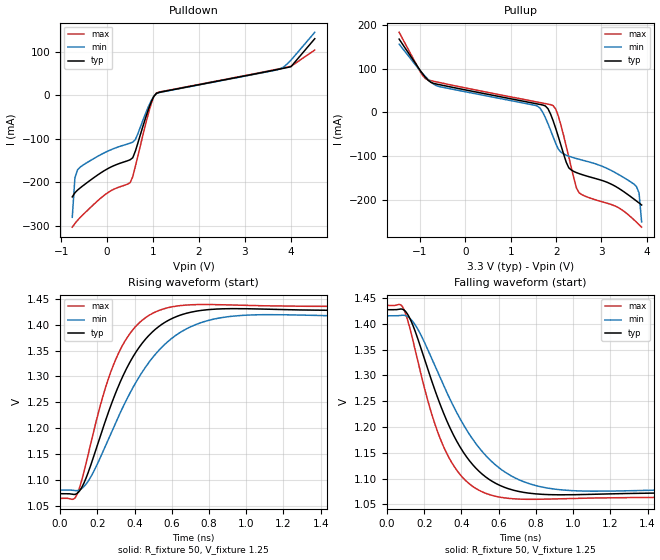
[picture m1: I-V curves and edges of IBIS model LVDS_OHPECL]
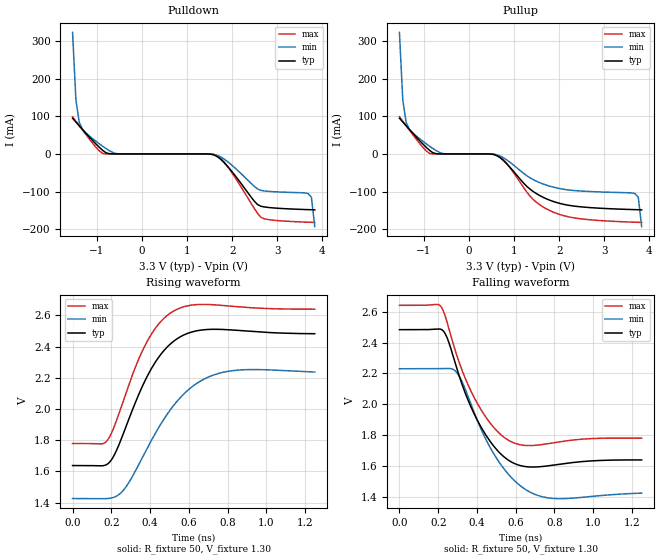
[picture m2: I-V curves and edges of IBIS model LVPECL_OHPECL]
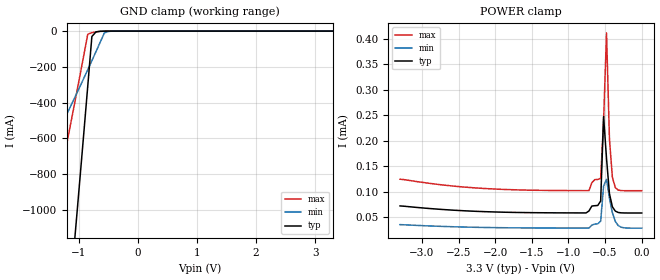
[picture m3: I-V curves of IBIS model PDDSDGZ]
|   This file is an IBIS representation of the   |
|   Integrated Device Technology Inc   |
|   IDT82P33714A   |
|   Synchronous Equipment Timing   |
|   Source for Synchronous Ethernet   |
[IBIS Ver]   4.1
[File name]   82p33714a.ibs
[File Rev]   0.5
|Rev 0.5
|08 Dec 2014
|Allegro Model Editor parse results, File passed: 0 errors, 33 warnings
|Rev 0.4
|06 Dec 2014
|pin 56 model name and pin name is NC because the pad is not bonded out
|Rev 0.3
|05 Dec 2014
|Added pin 73 as GND (ePad connection)
|Rev 0.2
|04 Dec 2014
|Updated pins 45 and 46
|Rev 0.1
|03 Dec 2014
|Original Model
[Date]   03 DEC 2014
[Source]   Originated at Integrated Device Technology, Inc.
[Notes]
No notes
[Disclaimer]
IDT hereby grants the user of this IBIS model a non-exclusive,
non-transferable license to use this IBIS model under the following terms.
Before using this IBIS model, the user should read this license.
If the user does not accept these terms,  the IBIS model should be
returned to IDT within 30 days.
   The user is granted this license only to use the IBIS model and
is not granted rights to sell, load, rent, lease or license the IBIS
model in whole or in part, or in modified form to anyone other than
user. User may modify the IBIS model to suit its specific
applications but rights to derivative works and such modifications
shall belong to IDT.
   This IBIS model is provided on an "AS IS" basis and IDT makes
absolutely no warranty with respect to the information contained
herein. IDT DISCLAIMS AND CUSTOMER WAIVES ALL WARRANTIES, EXPRESS
OR IMPLIED, INCLUDING WARRANTIES OF MERCHANTABILITY OR FITNESS FOR
A PARTICULAR PURPOSE. The entire risk as to quality and performance
is with the Customer. ACCORDINGLY, IN NO EVENT SHALL THE COMPANY BE
LIABLE FOR ANY DAMAGES, WHETHER IN CONTRACT OR TORT,INCLUDING ANY
LOST PROFITS OR OTHER INCIDENTAL, CONSEQUENTIAL, EXEMPLARY, OR
PUNITIVE DAMAGES ARISING OUT OF THE USE OR APPLICATION OF THE IBIS
model provided in this package. Further, IDT reserves the right to
make changes without notice to any product herein to improve
reliability, function, or design. IDT does not convey any license
under patent rights or any other intellectual property rights,
including those of third parties.
   IDT is not obligated to provide maintenance or support
for the licensed IBIS model.
[Copyright] Copyright 2014 by Integrated Device Technology, Inc.
[Component]   IDT82P33714A
[Manufacturer] Integrated Device Technology, Inc.
[Package]
|NLG 72
|   typ   min   max
R_pkg   0.14662   0.14662   0.14662
L_pkg   2.064e-9   2.064e-9   2.064e-9
C_pkg   3.399e-12   3.399e-12   3.399e-12
[Pin]   signal_name   model_name   R_pin   L_pin   C_pin
1   VC2   NC   159.1129532e-3  2.330616742e-9  290.6011e-15
2   VDDA   POWER   80.55656693e-3  1.627074523e-9  368.4314e-15
3   VDDA   POWER   82.37314399e-3  1.61436763e-9   359.8344e-15
4   VDDA   POWER   83.90273432e-3  1.632152529e-9  365.4028e-15
5   VDDA   POWER   88.16928499e-3  1.691978222e-9  379.0725e-15
6   OSCI   PDIDGZ   146.7372238e-3  2.417572968e-9  292.6019e-15
7   XO_FREQ0/LOS0   PDDSDGZ   133.245742e-3   2.24699185e-9   280.7049e-15
8   XO_FREQ1/LOS1   PDDSDGZ   124.3227716e-3  2.089820262e-9  264.6841e-15
9   XO_FREQ2/LOS2   PDDSDGZ   119.3648461e-3  1.952561307e-9  249.2576e-15
10   VDDA   POWER   67.96352653e-3  1.277137683e-9  316.527e-15
11   VDDA   POWER   124.3606471e-3  1.803394983e-9  258.8162e-15
12   VDDA   POWER   45.40697553e-3  1.045816154e-9  381.861e-15
13   VC1   NC   122.5820275e-3  1.79486331e-9   251.4324e-15
14   TMS   PDUSDGZ   117.199996e-3   1.881836464e-9  243.7828e-15
15   TRSTB   PDUSDGZ   117.9505235e-3  1.959346923e-9  249.952e-15
16   TCK   PDDSDGZ   124.0105416e-3  2.055224639e-9  260.0248e-15
17   TDI   PDUSDGZ   132.6063283e-3  2.195081403e-9  275.8995e-15
18   TDO   PDT02DGZ   139.0580983e-3  2.375490982e-9  254.5569e-15
19   VSSAO   GND   81.99029019e-3  1.941331922e-9  317.2106e-15
20   VDDAO   POWER   73.85343737e-3  1.662854677e-9  366.3893e-15
21   OUT4_POS   PECL_LVDS04 121.7311063e-3  1.941431983e-9  266.714e-15
22   OUT4_NEG   PECL_LVDS04 107.5226543e-3  1.73548545e-9   231.1601e-15
23   VSSAO   GND   55.50550232e-3  1.238142672e-9  269.1671e-15
24   VDDAO   POWER   51.03037114e-3  1.120699481e-9  265.15e-15
25   OUT3_POS   PECL_LVDS04 88.13552011e-3  1.429561675e-9  207.5597e-15
26   OUT3_NEG   PECL_LVDS04 84.21161109e-3  1.379390516e-9  197.1123e-15
27   VDDDO   POWER   46.76944028e-3  998.9182167e-9  232.0838e-15
28   OUT2   PDO08CDG   86.16174582e-3  1.377671438e-9  199.8731e-15
29   VDDDO   POWER   47.51781649e-3  996.4207054e-9  245.1067e-15
30   OUT1   PDO08CDG   92.05055036e-3  1.515185344e-9  202.4479e-15
31   IN1_POS   lvdspecl_rx 86.6701243e-3   1.443347965e-9  198.2298e-15
32   IN1_NEG   lvdspecl_rx 93.91076143e-3  1.549324015e-9  215.2678e-15
33   IN2_POS   lvdspecl_rx 104.444426e-3   1.718046615e-9  233.5331e-15
34   IN2_NEG   lvdspecl_rx 116.8021523e-3  1.932360839e-9  258.363e-15
35   IN3_POS   lvdspecl_rx 131.5182922e-3  2.179307422e-9  291.0504e-15
36   IN3_NEG   lvdspecl_rx 141.9756831e-3  2.439789828e-9  273.2442e-15
37   IN5   PDDSDGZ   140.0551623e-3  2.412978327e-9  247.8168e-15
38   IN4_POS   lvdspecl_rx 126.4230008e-3  2.142248554e-9  254.6755e-15
39   IN4_NEG   lvdspecl_rx 119.9314187e-3  2.029050584e-9  247.6935e-15
40   VDDD   POWER   117.0922381e-3  1.990478433e-9  243.7891e-15
41   IN6   PDDSDGZ   61.39234119e-3  1.45567977e-9   290.6114e-15
42   VDDD_1_8   POWER   62.64670293e-3  1.428642413e-9  280.9995e-15
43   FRSYNC_8K_1PPS   PDO04CDG   125.5118157e-3  2.091755546e-9  248.7724e-15
44   MFRSYNC_2K_1PPS   PDO04CDG   118.5182609e-3  2.032772465e-9  241.1773e-15
45   MPU_MODE0/I2CM_SDA   PDU02SDGZ   118.7248552e-3  2.079337927e-9  237.1947e-15
46   MPU_MODE1/I2CM_SCL   PDU02SDGZ   116.1434147e-3  2.040116685e-9  240.7992e-15
47   SDI/I2C_AD2/UART_RX   PDDSDGZ   113.9184373e-3  2.005672797e-9  243.2646e-15
48   CLKE/I2C_AD1   PDDSDGZ   114.7639065e-3  2.023372275e-9  243.911e-15
49   CS/I2C_AD0   PDUSDGZ   119.2670929e-3  2.063087241e-9  249.1366e-15
50   SCLK/I2C_SCL   PDDSDGZ   125.4625035e-3  2.170317538e-9  259.0128e-15
51   SDO/I2C_SDA/UART_TX   PDU02SDGZ   134.5129774e-3  2.297443305e-9  272.3048e-15
52   RSTB   PDUSDGZ   144.9448535e-3  2.469905075e-9  278.2184e-15
53   VDDD_1_8   POWER   73.18502347e-3  1.697897064e-9  321.7456e-15
54   DPLL3_LOCK   PDO02CDG   73.30587215e-3  1.805509644e-9  286.9406e-15
55   DPLL1_LOCK   PDO02CDG   131.2037581e-3  2.269971476e-9  249.9768e-15
56   NC   NC
57   INT_REQ   PDT02DGZ   111.9942974e-3  1.823787365e-9  244.1426e-15
58   MS/SL   PDUSDGZ   54.06374355e-3  1.208304195e-9  279.0375e-15
59   LOS3   PDDSDGZ   91.44979742e-3  1.501013847e-9  210.5244e-15
60   OUT10   PDO08CDG   88.55779602e-3  1.462256672e-9  201.0622e-15
61   OUT9   PDO08CDG   83.69588131e-3  1.389134256e-9  199.3806e-15
62   VDDD   POWER   47.94070401e-3  993.0254377e-9  238.4781e-15
63   OUT8   PDO08CDG   88.97797819e-3  1.387693063e-9  197.6827e-15
64   VDDDO   POWER   50.19081992e-3  1.056276793e-9  240.4795e-15
65   OUT7   PDO08CDG   91.25440696e-3  1.457201564e-9  206.4251e-15
66   VDDDO   POWER   55.34448696e-3  1.15702755e-9   257.2621e-15
67   OUT6_NEG   PECL_LVDS04 100.1273738e-3  1.588127846e-9  221.0412e-15
68   OUT6_POS   PECL_LVDS04 113.6333223e-3  1.762765097e-9  250.6782e-15
69   VDDAO   POWER   70.67244584e-3  1.428806307e-9  324.875e-15
70   OUT5_NEG   PECL_LVDS04 124.2699555e-3  1.951978145e-9  261.0113e-15
71   OUT5_POS   PECL_LVDS04 142.9203716e-3  2.168494279e-9  305.0693e-15
72   VDDAO   POWER   93.00146904e-3  1.898111852e-9  344.1775e-15
73   VSSAO   GND   81.99029019e-3  1.941331922e-9  317.2106e-15
[Diff Pin]   inv_pin   vdiff   tdelay_typ   tdelay_min   tdelay_max
|Inputs
 31   32   100mV   NA   NA   NA
 33   34   100mV   NA   NA   NA
 35   36   100mV   NA   NA   NA
 38   39   100mV   NA   NA   NA
|Outputs
 25   26   NA   0   0   0
 21   22   NA   0   0   0
 71   70   NA   0   0   0
 68   67   NA   0   0   0
[Model Selector] PECL_LVDS04
LVDS_OHPECL   3.3V LVDS Output Driver
LVPECL_OHPECL   3.3V LVPECL Output Driver
| Models and submodels in the file (11): LVDS_OHPECL (Output), LVPECL_OHPECL (Output_ECL), PDDSDGZ (Input), PDO08CDG (Output), PDO04CDG (Output), PDO02CDG (Output), PDUSDGZ (Input), lvdspecl_rx (Input), PDT02DGZ (3-state), PDU02SDGZ (I/O), PDIDGZ (Input)
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[Model]   LVDS_OHPECL
Model_type   Output
Polarity   Non-Inverting
|   typ   min   max
C_comp   2pF   1.5pF   2.5pF
Vmeas = 1.25V
Rref = 50
Cref = 0
Vref = 1.25V
|   typ   min   max
[Voltage range]   3.3V   3.135V   3.465V
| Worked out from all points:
|   slope of the pulldown table from 0 to 0.495 V, typ, clamps not added: 23.6 ohm
|   slope of the pullup table from 0 to 0.495 V, typ, clamps not added: 49.3 ohm
|   rising waveform, R_fixture 50, V_fixture 1.25: 20-80 % time 245ps typ, 304ps min, 193ps max; typ from 1.07 V to 1.43 V
|   falling waveform, R_fixture 50, V_fixture 1.25: 20-80 % time 245ps typ, 304ps min, 193ps max; typ from 1.43 V to 1.07 V
[Pulldown]
|Voltage   I (typ)   I (min)   I (max)
|Note, modeling breaks down at 250mA and above.  This is well beyond the functional   |
|operating range of the device.  Should this scenario occur, catastrophic failure and   |
|possible damage to the device and/or board is of higher concern than the I-V curve   |
|behavior.  The IBIS checker will flag currents in excess of 10A with warnings.  Lines   |
|with currents in excess of 0.35 A have been commented out.  The points still remain|
|available to the user if the user desires to use them.   |
|-2.84000e+00   -5.30688e+01   -4.60169e+01   -6.49561e+01
|-2.38000e+00   -4.07182e+01   -3.57367e+01   -4.91647e+01
|-1.92000e+00   -2.83653e+01   -2.54540e+01   -3.33724e+01
|-1.46000e+00   -1.60091e+01   -1.51695e+01   -1.75745e+01
|-1.00000e+00   -3.65295e+00   -4.88655e+00   -1.77315e+00
|-9.90000e-01   -3.38442e+00   -4.66309e+00   -1.42972e+00
|-9.32644e-01   -1.84442e+00   -3.38153e+00   -4.05588e-01
|-8.75287e-01   -5.22833e-01   -2.10025e+00   -3.26469e-01
|-8.17931e-01   -2.67482e-01   -8.21699e-01   -3.12033e-01
-760.6mV  -233mA     -279.7mA   -302.3mA
-703.2mV  -223.5mA   -189.3mA   -293.9mA
-645.9mV  -217.5mA   -171.1mA   -286.7mA
-14.94mV  -170mA     -129.6mA   -225.5mA
501.3mV   -147.9mA   -109.9mA   -200.6mA
558.6mV   -143.4mA   -107.5mA   -186.7mA
616mV     -128mA     -101.6mA   -163.1mA
960.1mV   -15.71mA   -12.63mA   -19.86mA
1.075V    4.077mA    3.606mA    4.898mA
3.771V    60mA       60.11mA    60.87mA
4.01V     65.35mA    80.22mA    66.12mA
4.528V    129.4mA    144mA      103.5mA
| 5.04600e+00   2.59994e-01   1.76348e+00   2.05360e-01
| 5.56400e+00   3.32161e+00   4.50935e+00   1.54088e+00
| 6.08200e+00   6.62030e+00   7.25691e+00   5.75525e+00
| 6.60000e+00   9.92114e+00   1.00065e+01   9.97217e+00
[Pullup]
|Voltage   I (typ)   I (min)   I (max)
|Note, modeling breaks down at 250mA and above.  This is well beyond the functional   |
|operating range of the device.  Should this scenario occur, catastrophic failure and   |
|possible damage to the device and/or board is of higher concern than the I-V curve   |
|behavior.  The IBIS checker will flag currents in excess of 10A with warnings.  Lines   |
|with currents in excess of 0.35 A have been commented out.  The points still remain|
|available to the user if the user desires to use them.   |
|-2.84000e+00   6.99085e+00   6.68991e+00   7.57174e+00
|-2.38000e+00   4.06132e+00   4.25024e+00   3.82819e+00
|-1.92000e+00   1.13336e+00   1.81188e+00   3.20303e-01
-1.46V    167mA      155.6mA    182.5mA
-875.3mV  79.39mA    80.95mA    76.56mA
-588.5mV  63.59mA    59.29mA    68.52mA
1.591V    19.2mA     14.2mA     23.52mA
1.82V     8.437mA    -25.7mA    18.9mA
1.935V    -19.25mA   -55.77mA   15.52mA
2.05V     -55.57mA   -83.85mA   -8.737mA
2.279V    -126.2mA   -99.7mA    -101.3mA
2.509V    -139.6mA   -106.9mA   -183.4mA
3.771V    -201.8mA   -168.9mA   -250.1mA
3.828V    -206.4mA   -183.2mA   -255.8mA
3.885V    -211.1mA   -249.6mA   -261.5mA
| 3.94264e+00   -2.16138e-01   -6.40744e-01   -2.67350e-01
| 4.00000e+00   -2.22049e-01   -1.86978e+00   -2.73217e-01
| 4.01000e+00   -2.23263e-01   -2.09313e+00   -2.74250e-01
| 4.52800e+00   -9.77564e+00   -1.36708e+01   -3.93552e+00
| 5.04600e+00   -2.36907e+01   -2.52521e+01   -2.17292e+01
| 5.56400e+00   -3.76023e+01   -3.68312e+01   -3.95166e+01
| 6.08200e+00   -5.15104e+01   -4.84070e+01   -5.72987e+01
| 6.60000e+00   -6.54191e+01   -5.99802e+01   -7.50835e+01
[Ramp]
|   typ   min   max
dV/dt_r   0.215/0.251n   0.204/0.312n   0.226/0.197n
dV/dt_f   0.858/0.18n   0.851/0.206n   0.863/0.152n
R_load =   50.0000
[Rising Waveform]
R_fixture = 50
V_fixture = 1.25   |Vcc_typ
V_fixture_min = 1.25 |Vcc_min
V_fixture_max = 1.25 |Vcc_max
C_fixture = 0.0p
| Time   typ   min   max
0s        1.073V     1.08V      1.064V
76.08ps   1.071V     1.079V     1.063V
114.1ps   1.084V     1.082V     1.096V
222.2ps   1.191V     1.148V     1.252V
296.3ps   1.266V     1.209V     1.331V
386.4ps   1.335V     1.275V     1.388V
496.5ps   1.386V     1.336V     1.422V
666.7ps   1.421V     1.39V      1.438V
882.9ps   1.431V     1.415V     1.439V
2ns       1.427V     1.415V     1.435V
[Falling Waveform]
R_fixture = 50
V_fixture = 1.25   |Vcc_typ
V_fixture_min = 1.25 |Vcc_min
V_fixture_max = 1.25 |Vcc_max
C_fixture = 0.0p
| Time   typ   min   max
0s        1.427V     1.415V     1.435V
76.08ps   1.428V     1.416V     1.436V
114.1ps   1.416V     1.413V     1.403V
222.2ps   1.309V     1.347V     1.247V
296.3ps   1.234V     1.287V     1.168V
386.4ps   1.165V     1.22V      1.111V
496.5ps   1.114V     1.159V     1.077V
666.7ps   1.079V     1.106V     1.061V
882.9ps   1.069V     1.081V     1.061V
2ns       1.073V     1.08V      1.064V
[Model]   LVPECL_OHPECL
Model_type   Output_ECL
Polarity   Non-Inverting
|   typ   min   max
C_comp   2pF   1.5pF   2.5pF
Vmeas = 2.08V
Rref = 50
Cref = 0
Vref = 1.3V
|   typ   min   max
[Voltage range]   3.3V   3.135V   3.465V
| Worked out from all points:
|   rising waveform, R_fixture 50, V_fixture 1.30: 20-80 % time 183ps typ, 239ps min, 167ps max; typ from 1.64 V to 2.48 V
|   falling waveform, R_fixture 50, V_fixture 1.30: 20-80 % time 166ps typ, 189ps min, 167ps max; typ from 2.48 V to 1.64 V
[Pulldown]
|Voltage   I (typ)   I (min)   I (max)
|Note, modeling breaks down at 250mA and above.  This is well beyond the functional   |
|operating range of the device.  Should this scenario occur, catastrophic failure and   |
|possible damage to the device and/or board is of higher concern than the I-V curve   |
|behavior.  The IBIS checker will flag currents in excess of 10A with warnings.  Lines   |
|with currents in excess of 0.35 A have been commented out.  The points still remain|
|available to the user if the user desires to use them.   |
|-3.04000e+00   8.13628e+00   7.40568e+00   9.05264e+00
|-2.78000e+00   6.48842e+00   6.17138e+00   6.94615e+00
|-2.52000e+00   4.84065e+00   4.93719e+00   4.83974e+00
|-2.26000e+00   3.19294e+00   3.70309e+00   2.73339e+00
|-2.00000e+00   1.54529e+00   2.46908e+00   6.27077e-01
|-1.99000e+00   1.48192e+00   2.42162e+00   5.48040e-01
|-1.91540e+00   1.00920e+00   2.06758e+00   1.98610e-01
|-1.84080e+00   5.37180e-01   1.71354e+00   1.48402e-01
|-1.76621e+00   2.09338e-01   1.35951e+00   1.34910e-01
|-1.69161e+00   1.23802e-01   1.00548e+00   1.22822e-01
|-1.61701e+00   1.05710e-01   6.51459e-01   1.10791e-01
-1.542V   94.94mA    323.2mA    98.78mA
-1.468V   84.75mA    142.9mA    86.78mA
-1.393V   74.65mA    83.42mA    74.82mA
-1.095V   35.36mA    40.48mA    28.07mA
-871mV    9.149mA    20.06mA    1.232mA
-572.6mV  4.108uA    982.2uA    950.7nA
1.665V    -6.941mA   -3.619mA   -4.645mA
1.964V    -42.69mA   -27.19mA   -45.05mA
2.635V    -138.9mA   -96.87mA   -168.4mA
3.679V    -147.9mA   -105.1mA   -181.4mA
3.754V    -148.2mA   -115mA     -181.7mA
3.829V    -148.6mA   -193mA     -182mA
| 3.90322e+00   -1.49228e-01   -8.48432e-01   -1.82298e-01
| 3.97782e+00   -1.50944e-01   -2.34373e+00   -1.82574e-01
| 4.05241e+00   -1.56521e-01   -3.83983e+00   -1.82884e-01
| 4.12701e+00   -2.02437e-01   -5.33650e+00   -1.83452e-01
| 4.20161e+00   -9.28214e-01   -6.83362e+00   -1.85046e-01
| 4.27621e+00   -2.92725e+00   -8.33107e+00   -1.88918e-01
| 4.35080e+00   -4.92706e+00   -9.82879e+00   -2.02110e-01
| 4.42540e+00   -6.92744e+00   -1.13267e+01   -4.86879e-01
| 4.50000e+00   -8.92826e+00   -1.28248e+01   -2.83371e+00
| 4.51000e+00   -9.19650e+00   -1.30256e+01   -3.17645e+00
| 4.92800e+00   -2.04120e+01   -2.14217e+01   -1.75120e+01
| 5.34600e+00   -3.16289e+01   -2.98181e+01   -3.18527e+01
| 5.76400e+00   -4.28445e+01   -3.82136e+01   -4.61922e+01
| 6.18200e+00   -5.40593e+01   -4.66077e+01   -6.05302e+01
| 6.60000e+00   -6.52756e+01   -5.50006e+01   -7.48692e+01
[Pullup]
|Voltage   I (typ)   I (min)   I (max)
|Note, modeling breaks down at 250mA and above.  This is well beyond the functional   |
|operating range of the device.  Should this scenario occur, catastrophic failure and   |
|possible damage to the device and/or board is of higher concern than the I-V curve   |
|behavior.  The IBIS checker will flag currents in excess of 10A with warnings.  Lines   |
|with currents in excess of 0.35 A have been commented out.  The points still remain|
|available to the user if the user desires to use them.   |
|-3.04000e+00   8.13628e+00   7.40568e+00   9.05264e+00
|-2.78000e+00   6.48842e+00   6.17138e+00   6.94615e+00
|-2.52000e+00   4.84065e+00   4.93719e+00   4.83974e+00
|-2.26000e+00   3.19294e+00   3.70309e+00   2.73339e+00
|-2.00000e+00   1.54529e+00   2.46908e+00   6.27077e-01
|-1.99000e+00   1.48192e+00   2.42162e+00   5.48040e-01
|-1.91540e+00   1.00920e+00   2.06758e+00   1.98610e-01
|-1.84080e+00   5.37180e-01   1.71354e+00   1.48402e-01
|-1.76621e+00   2.09338e-01   1.35951e+00   1.34910e-01
|-1.69161e+00   1.23802e-01   1.00548e+00   1.22822e-01
|-1.61701e+00   1.05710e-01   6.51459e-01   1.10791e-01
-1.542V   94.94mA    323.2mA    98.78mA
-1.468V   84.75mA    142.9mA    86.78mA
-1.393V   74.65mA    83.42mA    74.82mA
-1.095V   35.36mA    40.48mA    28.07mA
-871mV    9.149mA    20.06mA    1.232mA
-572.6mV  4.135uA    982.3uA    950.9nA
620.9mV   -4.811mA   -2.487mA   -2.686mA
1.441V    -101.4mA   -69.34mA   -123mA
1.964V    -129.9mA   -90.95mA   -159mA
3.679V    -148mA     -105.2mA   -181.5mA
3.754V    -148.3mA   -115.1mA   -181.8mA
3.829V    -148.6mA   -193.1mA   -182.1mA
| 3.90322e+00   -1.49284e-01   -8.48518e-01   -1.82336e-01
| 3.97782e+00   -1.50988e-01   -2.34381e+00   -1.82600e-01
| 4.05241e+00   -1.56557e-01   -3.83989e+00   -1.82901e-01
| 4.12701e+00   -2.02464e-01   -5.33656e+00   -1.83462e-01
| 4.20161e+00   -9.28235e-01   -6.83367e+00   -1.85048e-01
| 4.27621e+00   -2.92726e+00   -8.33112e+00   -1.88915e-01
| 4.35080e+00   -4.92707e+00   -9.82883e+00   -2.02102e-01
| 4.42540e+00   -6.92745e+00   -1.13267e+01   -4.86867e-01
| 4.50000e+00   -8.92826e+00   -1.28248e+01   -2.83369e+00
| 4.51000e+00   -9.19650e+00   -1.30257e+01   -3.17644e+00
| 4.92800e+00   -2.04120e+01   -2.14217e+01   -1.75119e+01
| 5.34600e+00   -3.16288e+01   -2.98182e+01   -3.18526e+01
| 5.76400e+00   -4.28444e+01   -3.82136e+01   -4.61920e+01
| 6.18200e+00   -5.40590e+01   -4.66077e+01   -6.05298e+01
| 6.60000e+00   -6.52749e+01   -5.50006e+01   -7.48682e+01
[Ramp]
|   typ   min   max
dV/dt_r   0.525/0.194n   0.496/0.247n   0.537/0.177n
dV/dt_f   0.537/0.183n   0.507/0.204n   0.549/0.185n
R_load =   50.0000
[Rising Waveform]
R_fixture = 50
V_fixture = 1.30   | VCC_typ - 2V
V_fixture_max = 1.465   | VCC_max - 2V
V_fixture_min = 1.135   | VCC_min - 2V
C_fixture = 0.0p
| Time   typ   min   max
0s        1.637V     1.426V     1.779V
180.2ps   1.647V     1.426V     1.8V
216.5ps   1.708V     1.435V     1.892V
266.5ps   1.856V     1.485V     2.07V
376.6ps   2.188V     1.728V     2.414V
446.7ps   2.336V     1.886V     2.549V
524.3ps   2.437V     2.027V     2.63V
639.4ps   2.501V     2.163V     2.67V
772ps     2.51V      2.234V     2.665V
1.25ns    2.483V     2.237V     2.64V
[Falling Waveform]
R_fixture = 50
V_fixture = 1.30   | VCC_typ - 2V
V_fixture_max = 1.465   | VCC_max - 2V
V_fixture_min = 1.135   | VCC_min - 2V
C_fixture = 0.0p
| Time   typ   min   max
0s        2.483V     2.23V      2.641V
207.7ps   2.487V     2.231V     2.642V
242.7ps   2.44V      2.232V     2.545V
289ps     2.262V     2.215V     2.344V
349.1ps   2.042V     2.067V     2.14V
416.7ps   1.862V     1.851V     1.973V
568.1ps   1.632V     1.538V     1.762V
663.2ps   1.594V     1.437V     1.732V
769.5ps   1.601V     1.392V     1.745V
1.25ns    1.638V     1.423V     1.78V
|   Model PDDSDGZ
[Model]  PDDSDGZ
Model_type Input
Polarity   Non-Inverting
Vinl =   0.8000V
Vinh =   2.0000V
C_comp   2.6812pF   2.6701pF   2.6826pF
[Temperature Range]   25.0000   0.1250k   -40.0000
[Voltage Range]   3.3000V   3.0000V   3.6000V
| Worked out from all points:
|   GND clamp passes 1 mA (typ) near -0.64 V on its own axis
[GND_clamp]
|Voltage   I(typ)   I(min)   I(max)
-3.3V     -8.473A    -1.702A    -3.67A
-2.25V    -5.322A    -1.128A    -2.26A
-2.18V    -5.094A    -1.087A    -2.158A
-1.55V    -2.941A    -695.2mA   -1.195A
-1.48V    -2.689A    -649.4mA   -1.083A
-1.06V    -1.126A    -365mA     -383.4mA
-850mV    -308.3mA   -216.3mA   -17.65mA
-780mV    -30.2mA    -165.7mA   -8.739mA
-710mV    -4.257mA   -114.6mA   -4.589mA
-570mV    -195.9uA   -10.81mA   -435.6uA
-500mV    -58.31uA   -1.732mA   -98.01uA
3.3V      57.9uA     29.96uA    101.7uA
[POWER_clamp]
|Voltage   I(typ)   I(min)   I(max)
-3.3V     71.8uA     35.04uA    124.4uA
-2.16V    60.67uA    29.52uA    106.2uA
-720mV    61.92uA    28.24uA    101.9uA
-680mV    71.62uA    34.23uA    117.6uA
-560mV    81.4uA     41.85uA    126.2uA
-520mV    247.4uA    111uA      238.4uA
-480mV    165.3uA    124.1uA    412.1uA
-440mV    95.84uA    86.88uA    203.4uA
-400mV    70.17uA    58.44uA    128.3uA
-360mV    61.63uA    41.31uA    107.7uA
-320mV    58.98uA    33.21uA    103uA
0V        57.91uA    28.11uA    101.8uA
